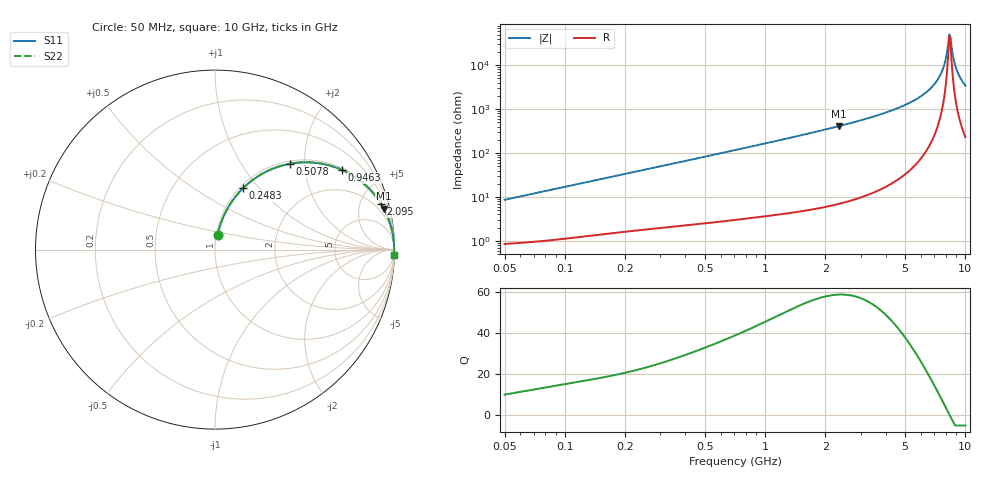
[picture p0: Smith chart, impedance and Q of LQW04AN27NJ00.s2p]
!Murata Part Number: LQW04AN27NJ00
!These Parameters are Measured in Series Mode Connection
!  o--[Z]--o
!Port1  Port2
!  o-------o
!Freq. Start=50[MHz] Stop=10[GHz], 401[Steps]
# Hz S RI R 50
!Freq.(Hz)	S 11(Real)	S 11(Imag)	S 21(Real)	S 21(Imag)	S 12(Real)	S 12(Imag)	S 22(Real)	S 22(Imag)
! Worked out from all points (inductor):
!   401 points, 50 MHz to 10 GHz, reference 50 ohm
!   read as one part in series: L = 27.2 nH near 51.34 MHz
!   highest Q = 58.9 at 2.329 GHz (marker M1), where L = 27.9 nH
!   self-resonance near 8.307 GHz
!   S11 on the Smith chart (normalised r, x): 50 MHz: 1.02, +0.17; 248.3 MHz: 1.04, +0.83; 507.8 MHz: 1.05, +1.68; 946.3 MHz: 1.07, +3.13; 2.095 GHz: 1.12, +7.25; 10 GHz: 6, -69
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5e7  0.0156 0.0837  0.9844 -0.0837  0.9844 -0.0837  0.0156 0.0837
1.214486e8  0.0514 0.1927  0.9486 -0.1927  0.9486 -0.1927  0.0514 0.1927
2.483314e8  0.1569 0.3427  0.8431 -0.3427  0.8431 -0.3427  0.1569 0.3427
2.949953e8  0.2032 0.383  0.7968 -0.383  0.7968 -0.383  0.2032 0.383
5.077742e8  0.4154 0.478  0.5846 -0.478  0.5846 -0.478  0.4154 0.478
7.071068e8  0.5746 0.4817  0.4254 -0.4817  0.4254 -0.4817  0.5746 0.4817
9.463279e8  0.7059 0.4445  0.2941 -0.4445  0.2941 -0.4445  0.7059 0.4445
1.717543e9  0.8902 0.3039  0.1098 -0.3039  0.1098 -0.3039  0.8902 0.3039
2.095058e9  0.9255 0.2542  0.0745 -0.2542  0.0745 -0.2542  0.9255 0.2542
2.329253e9  0.9401 0.2289  0.0599 -0.2289  0.0599 -0.2289  0.9401 0.2289
4.171863e9  0.9853 0.1101  0.0147 -0.1101  0.0147 -0.1101  0.9853 0.1101
5.657692e9  0.9944 0.0596  0.00556 -0.0596  0.00556 -0.0596  0.9944 0.0596
6.901252e9  0.9973 0.029  0.00271 -0.029  0.00271 -0.029  0.9973 0.029
7.672705e9  0.998 0.0129  0.002 -0.0129  0.002 -0.0129  0.998 0.0129
7.878683e9  0.9981 0.00889  0.00191 -0.00889  0.00191 -0.00889  0.9981 0.00889
8.198065e9  0.9982 0.00281  0.00184 -0.00281  0.00184 -0.00281  0.9982 0.00281
8.307378e9  0.9982 0.000765  0.00184 -0.000765  0.00184 -0.000765  0.9982 0.000765
8.530394e9  0.9981 -0.00333  0.00185 0.00333  0.00185 0.00333  0.9981 -0.00333
8.876195e9  0.9981 -0.00955  0.00194 0.00955  0.00194 0.00955  0.9981 -0.00955
9.114482e9  0.9979 -0.0137  0.00206 0.0137  0.00206 0.0137  0.9979 -0.0137
9.610418e9  0.9976 -0.0223  0.0024 0.0223  0.0024 0.0223  0.9976 -0.0223
1e10  0.9972 -0.0289  0.00279 0.0289  0.00279 0.0289  0.9972 -0.0289
